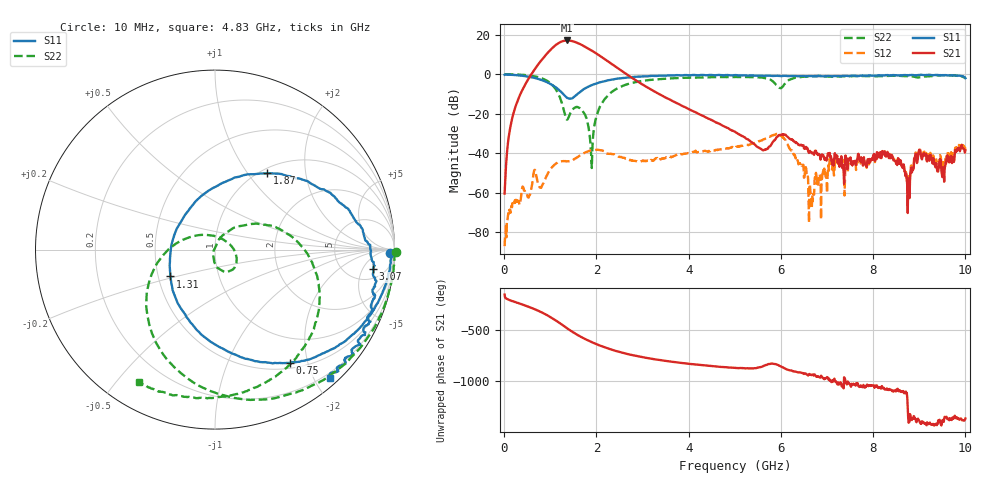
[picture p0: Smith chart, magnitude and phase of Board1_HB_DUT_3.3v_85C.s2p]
! Created Tue May 27 14:06:45 2025
# hz S ma R 50
! 2 Port Network Data from SP1.SP block
! freq  magS11  angS11  magS21  angS21  magS12  angS12  magS22  angS22
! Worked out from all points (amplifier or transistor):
!   1000 points, 10 MHz to 10 GHz, reference 50 ohm
!   highest |S21| = 17.2 dB at 1.36 GHz (marker M1)
!   |S21| within 3 dB of that: 1.084 GHz to 1.741 GHz (656.7 MHz wide, 46.5 % of centre)
!   unconditionally stable (mu >= 1): 59.24 MHz to 61.34 MHz; 90.87 MHz to 103 MHz; 116.5 MHz to end of sweep
!   at 1.67 GHz: K = 8.22, MAG = 15.8 dB, |S12| = -40.8 dB
!   at 5.01 GHz: K = 21.60, MAG = -12.5 dB, |S12| = -37.0 dB
!   at 10 GHz: K = 337.59, MAG = -29.0 dB, |S12| = -37.1 dB
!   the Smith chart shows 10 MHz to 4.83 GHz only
!   S11 on the Smith chart (normalised r, x): 10 MHz: 53, -36; 750 MHz: 0.58, -1.71; 1.31 GHz: 0.58, -0.19; 1.87 GHz: 1.07, +1.24; 3.07 GHz: 8, -8; 4.83 GHz: 0.12, -2.22
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1e7  0.9743 -1.0  0.0009407 -147.2  4.347e-05 85.1  1.006 -0.8
2.2e8  0.9608 -15.3  0.1205 140.8  0.0005403 75.6  0.9932 -20.3
7.5e8  0.7567 -56.5  1.853 51.0  0.001519 69.6  0.8415 -80.9
9.3e8  0.6302 -74.6  3.378 10.6  0.002745 118.3  0.684 -110.6
1.09e9  0.4953 -96.1  5.185 -32.5  0.005071 101.1  0.464 -145.3
1.19e9  0.3973 -114.7  6.305 -62.8  0.005922 87.6  0.291 -173.8
1.31e9  0.2895 -148.9  7.138 -101.4  0.006237 76.1  0.104 127.6
1.36e9  0.2552 -169.3  7.235 -117.3  0.006215 73.0  0.07076 71.3
1.51e9  0.261 125.5  6.788 -162.3  0.006907 74.8  0.1364 -28.6
1.68e9  0.382 81.3  5.582 153.3  0.009347 66.8  0.1278 -69.7
1.87e9  0.5149 55.7  4.189 110.9  0.01148 47.6  0.01855 -123.0
2.23e9  0.695 28.7  2.219 46.4  0.00977 11.8  0.2727 32.1
2.57e9  0.8032 10.8  1.174 -0.2  0.007624 0.7  0.5104 -1.8
3.07e9  0.8886 -7.0  0.4927 -48.4  0.006227 10.3  0.6993 -37.5
3.34e9  0.9161 -15.7  0.3238 -68.5  0.0067 10.3  0.7529 -52.8
4.83e9  0.9605 -48.3  0.04402 -142.6  0.0134 -7.9  0.8501 -120.0
5.01e9  0.9588 -52.1  0.03437 -147.5  0.01412 -12.4  0.855 -126.8
5.98e9  0.9024 -72.2  0.02859 -129.9  0.02843 -100.9  0.4506 -152.0
6.67e9  0.8996 -92.4  0.009928 143.6  0.0003881 137.8  0.8934 -157.4
8.34e9  0.9317 -135.4  0.007498 -5.8  0.007828 -11.6  0.9134 167.0
8.75e9  0.9486 -142.7  0.0003019 -173.1  0.0004311 115.4  0.8999 158.5
1e10  0.8001 -161.7  0.01184 75.1  0.01403 71.5  0.83 145.2
